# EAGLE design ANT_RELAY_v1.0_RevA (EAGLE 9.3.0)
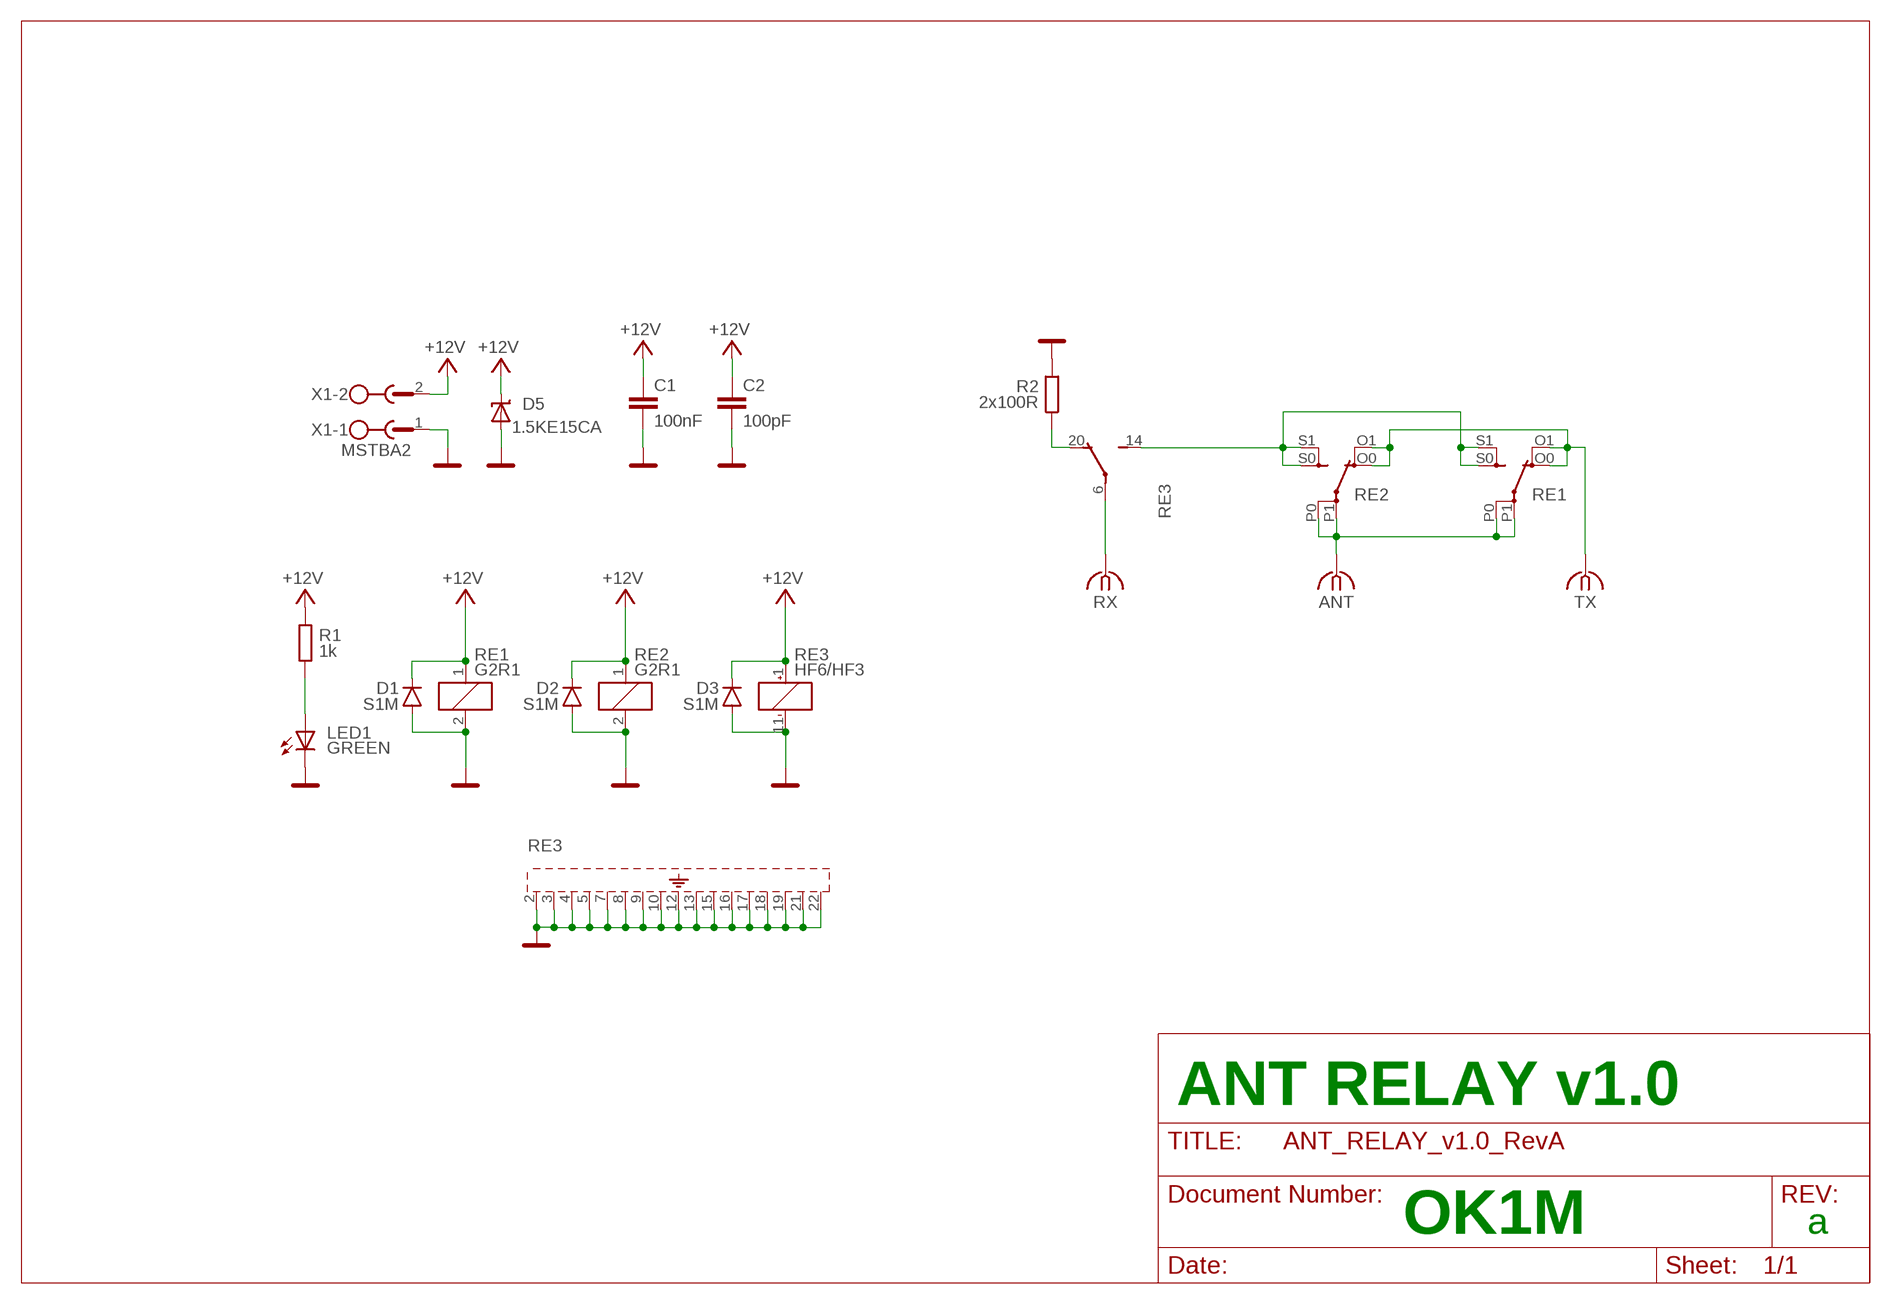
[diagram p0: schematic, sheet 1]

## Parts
ANT  N-180  [N-180]
C1  100nF  C-EUC0805  [C0805]
C2  100pF  C-EUC0805  [C0805]
D1  S1M  [SMA]
D2  S1M  [SMA]
D3  S1M  [SMA]
D5  1.5KE15CA  TRANSILDO201-15  [DO201-15]
LED1  GREEN  LED3MM  [LED3MM]
R1  1k  R-EU_M0805  [M0805]
R2  2x100R  R-EU_M1206  [M1206]
RE1  G2R1  G2RE  [G2RE]
RE2  G2R1  G2RE  [G2RE]
RE3  HF6/HF3  HF6-56+  [HF6-56]
RX  N-180  [N-180]
TX  N-180  [N-180]
X1  MSTBA2  [MSTBA2]

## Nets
+12V: C1.1 C2.1 D1.C D2.C D3.C D5.C R1.2 RE1.1 RE2.1 RE3.1 X1.2
ANT: ANT.1 RE1.P0(2:P) RE1.P1(2:P) RE2.P0(2:P) RE2.P1(2:P)
GND: C1.2 C2.2 D1.A D2.A D3.A D5.A LED1.K(C) R2.2 RE1.2 RE2.2 RE3.2 RE3.3 RE3.4 RE3.5 RE3.7 RE3.8 RE3.9 RE3.10 RE3.11 RE3.12 RE3.13 RE3.15 RE3.16 RE3.17 RE3.18 RE3.19 RE3.21 RE3.22 X1.1
N$2: RE3.6 RX.1
N$5: R2.1 RE3.20
N$20: LED1.A R1.1
N$30: RE1.S0(2:S) RE1.S1(2:S) RE2.S0(2:S) RE2.S1(2:S) RE3.14
TX: RE1.O0(2:O) RE1.O1(2:O) RE2.O0(2:O) RE2.O1(2:O) TX.1

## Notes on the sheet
- ANT RELAY v1.0
- OK1M | a

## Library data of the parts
ANT RX TX = #my:N-180
C1 C2 = rcl:C-EU: CAPACITOR, European symbol; SPICEPREFIX: C
D1-D3 = diode:S1M
D5 = #Marek:TRANSIL: TRANSIL
LED1 = led:LED: LED
R1 R2 = rcl:R-EU_: RESISTOR, European symbol
RE1 RE2 = relay:G2RE: RELAY 1 x switch, high current, Omron; OC_FARNELL: unknown; OC_NEWARK: unknown
RE3 = #hf6-56:HF6-56+
X1 = con-phoenix-508:MSTBA2: PHOENIX; MF: FARNELL; MPN: 1757242; OC_FARNELL: 3705171; OC_NEWARK: 71C4161

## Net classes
0 default: width 0.203 mm, drill 0.406 mm, clearance 0.203 mm

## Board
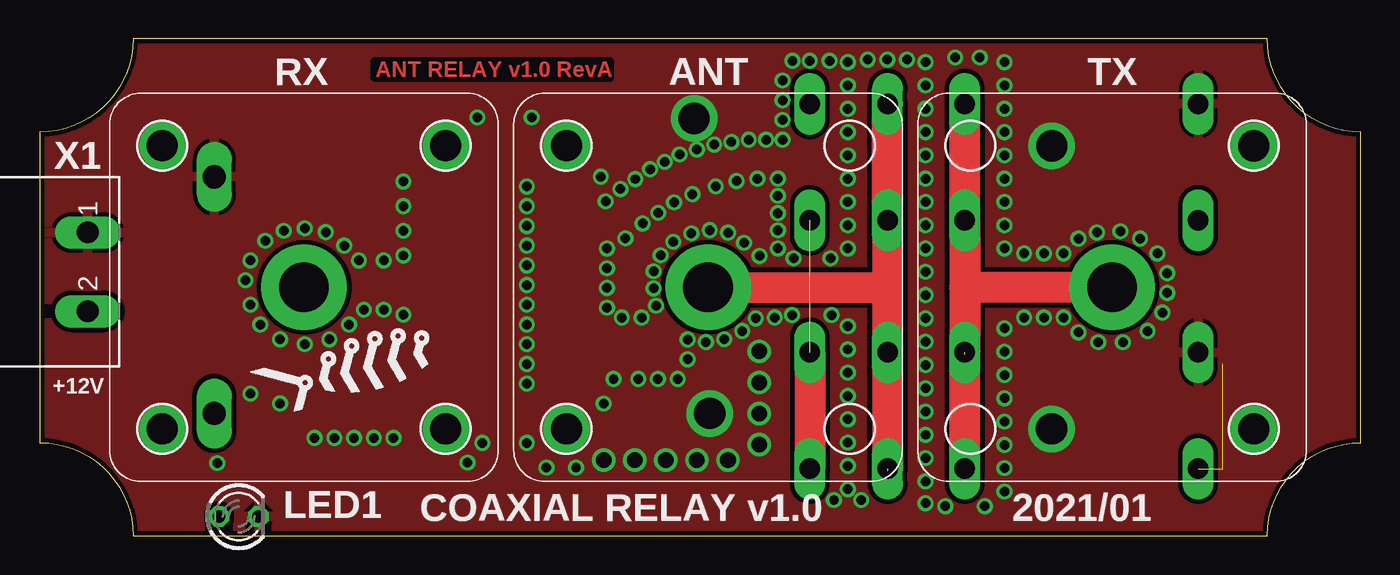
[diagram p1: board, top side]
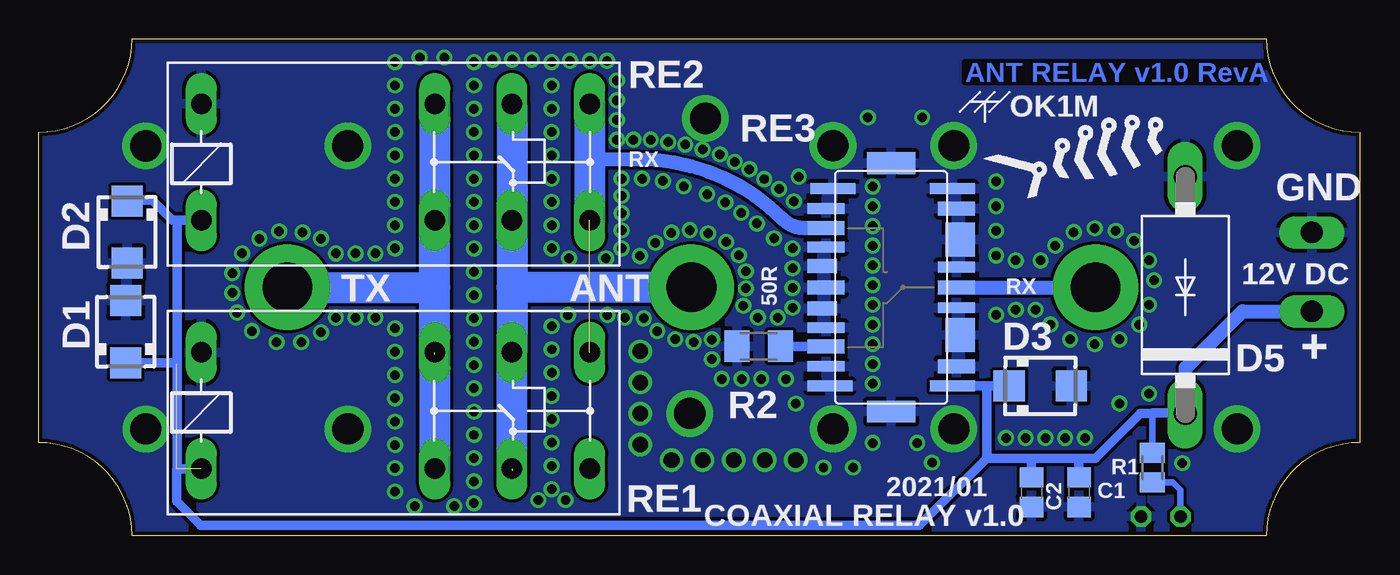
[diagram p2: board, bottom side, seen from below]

Size 85 x 32 mm. Coordinates in mm from the lower left corner, seen from the top.
Outline: 6,0 79,0 arc-90 85,6 85,26 arc-90 79,32 6,32 arc-90 0,26 0,6 arc-90 6,0
Copper layers (1*16): Top 0.035mm / dielectric 1.5mm / Bottom 0.035mm
Design rules "default *": minimum track width 10mil, minimum drill 24mil, track to track 8mil, track to pad 8mil, pad to pad 8mil, via to via 8mil, smd to smd 8mil, copper to edge 10mil, drill to drill 8mil, minimum pad ring 10mil, minimum via ring 8mil, stop-mask expansion 4mil, vias tented up to drill 0.7mm, thermal gap 10mil

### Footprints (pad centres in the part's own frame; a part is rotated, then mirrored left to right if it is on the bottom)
N-180 = drill 3.2 pad 5.5: 1 0,0
C0805 = smd 1.3 x 1.5: 1 -0.95,0; 2 0.95,0
SMA = smd 2 x 2: A 2,0; C -2,0
DO201-15 = drill 1.499 long: A 7.62,0; C -7.62,0
LED3MM = drill 0.813 octagon: A -1.27,0; K 1.27,0
M0805 = smd 1.3 x 1.6: 1 -0.95,0; 2 0.95,0
M1206 = smd 1.6 x 2: 1 -1.4,0; 2 1.4,0
G2RE = drill 1.321 long: 1 -2.54,-3.683; 2 -2.54,3.81; O0 12.471,-3.683; O1 12.471,3.81; P0 17.45,-3.683; P1 17.45,3.81; S0 22.454,-3.683; S1 22.454,3.81
HF6-56 = smd 0.7 x 2.9: 1 -6.35,-3.95; 11 6.35,-3.95; 12 6.35,3.75; 22 -6.35,3.95 | smd 0.9 x 2.4: 2 -5.08,-4.2; 6 0,-4.2; 10 5.08,-4.2; 14 3.81,4.2; 17 0,4.2; 20 -3.81,4.2 | smd 2.2 x 1.9: 3 -3.075,-4.45; 8 3.075,-4.45 | smd 1.4 x 3.1: 4 -8,0; 9 8,0 | smd 0.7 x 2.4: 5 -1.317,-4.2; 7 1.317,-4.2; 13 5.08,4.2; 15 2.6,4.2; 19 -2.6,4.2; 21 -5.08,4.2 | smd 0.9 x 1.9: 16 1.375,4.45; 18 -1.375,4.45
MSTBA2 = drill 1.397 long: 1 -2.54,5.08; 2 2.54,5.08

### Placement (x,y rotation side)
ANT  43,16 0 top
C1  18.06,2.81 270 bottom
C2  21.12,2.81 270 bottom
D1  79.41,13.14 90 bottom
D2  79.32,19.56 270 bottom
D3  20.56,9.65 0 bottom
D5  11.22,15.5 90 bottom
LED1  12.8,1.24 0 top
R1  13.34,4.39 90 bottom
R2  38.67,12.21 180 bottom
RE1  72,8 0 bottom
RE2  72,24 0 bottom
RE3  30.15,16 90 bottom
RX  17,16 0 top
TX  69,16 0 top
U$1  [RYBICKA_12MM]  20.95,10.79 0 top
U$2  [RYBICKA_12MM]  16.75,24.53 0 bottom
X1  -2,17 270 top

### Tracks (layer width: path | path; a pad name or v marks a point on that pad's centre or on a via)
+12V  (2 unrouted)
  Bottom 0.406: R1.2 13.34,7.87 13.34,7.88 | D5.C 11.25,7.91 13.3,7.91
  Bottom 0.61: RE3.1 24,9.65 | 24,9.65 D3.C | RE2.1 76.09,20.32 | 76.09,20.32 76.4,20.32 77.71,21.62 D2.C | RE1.1 76.09,4.32 76.09,20.32 | D1.C 76.2,11.14 76.12,11.06 | 24,9.65 24,5 | 18.1,5 17,5 14.12,7.88 13.34,7.88 13.3,7.91 11.19,7.91 | 18.1,5 21.27,5 | 21.27,5 24,5 | 24,5 28.32,0.68 74.57,0.68 76.12,2.23 76.12,4.32 | C1.1 18.06,4.96 18.1,5 | C2.1 21.12,4.84 21.27,5
  Bottom 0.9: 11.19,7.91 11.19,10.81 7.54,14.46 X1.2
ANT  (1 unrouted)
  Top 2: 54.55,16 RE2.P0 RE2.P1 | 54.55,16 RE1.P1 RE1.P0 | ANT.1 54.55,16
  Bottom 2: 54.55,16 54.55,20.19 RE2.P0 54.55,27.68 | 54.55,16 RE1.P1 | 54.55,16 ANT.1 54.55,16 | 54.55,4.19 54.55,11.68
GND  (via drill 0.61, 1, 2)
  other vias: 57,29 57,30.5 57,27.5 57,26 57,24.5 57,23 57,21.5 57,20 57,18.5 57,17 57,15.5 57,14 57,12.5 57,11 57,9.5 57,8 57,6.5 57,5 57,3.5 57,2.1 52,29 52,30.5 52,27.5 52,26 52,24.5 52,23 52,21.5 52,20 52,18.5 47.5,18.5 46.32,18.02 45.32,18.86 44.29,19.52 43.11,19.68 52,12 52,13.5 52,10.5 52,9 52,7.5 52,6 52,4.5 52,3 41.93,19.48 40.77,18.93 39.95,18.06 39.5,17.04 41.68,12.63 42.87,12.48 44.05,12.66 45.21,13.18 46.07,14 36.5,18.5 38.79,20.11 39.79,20.79 40.82,21.48 42,22 43.5,22.5 44.84,22.84 46.18,23 47.5,23 37.68,19.16 36.41,21.54 37.37,22.33 38.32,22.97 39.27,23.6 40.22,24.08 41.17,24.56 42.29,24.87 43.4,25.19 44.51,25.35 45.62,25.51 46.73,25.51 47.8,25.51 47.8,26.78 47.8,28.05 47.8,29.32 48.44,30.59 49.55,30.59 50.82,30.59 47.5,21.89 47.5,20.78 47.5,19.67 39.5,15.93 39.66,14.82 36.5,17.23 36.5,15.96 36.5,14.69 37.45,14.05 38.72,14.05 47.3,14.05 50.95,14.21 50.89,17.86 48.51,17.86 54.54,30.66 53.27,30.66 55.81,30.66 48.41,14.21 51.1,2.31 52.85,2.31 11.42,4.69 36.09,23.13 31.33,22.49 31.33,21.22 31.33,19.95 31.33,18.68 31.33,17.41 31.33,16.14 31.33,14.87 31.33,13.6 31.33,12.33 31.33,11.06 31.33,9.79 41.68,11.37 41.05,10.1 39.78,10.1 38.51,10.1 36.92,10.1 36.28,8.51 7.88,25.13 26.12,25.12 33.89,25.13 26.12,6.88 33.89,6.88 78.12,25.11 78.11,6.88 7.88,6.88 46.29,11.87 46.29,9.87 46.29,7.87 46.29,5.87 44.29,4.87 42.29,4.87 40.29,4.87 38.29,4.87 36.29,4.87 62.08,11.86 62.08,13.36 62.08,10.36 62.08,8.86 62.08,7.36 62.08,5.86 62.08,4.36 62.08,2.85 62.08,29 62.08,30.5 62.08,27.5 62.08,26 62.08,24.5 62.08,23 62.08,21.5 62.08,20 62.08,18.5 63.35,18.18 65.89,18.18 64.62,18.18 63.35,14.05 64.62,14.05 65.89,14.05 66.84,13.1 68.11,12.47 69.7,12.47 71.29,13.18 72.24,14.37 72.56,15.64 72.56,16.91 71.92,18.18 70.81,19.14 69.54,19.61 68.03,19.53 66.84,19.14 60.81,1.9 58.27,1.9 60.49,30.8 58.91,30.8 28.16,26.94 31.65,26.94 23.39,22.81 23.39,21.22 23.39,19.64 23.39,18.05 23.39,14.24 22.12,17.73 20.54,17.73 19.59,18.68 18.39,19.56 17.05,19.79 15.7,19.64 14.51,19 13.55,17.73 13.23,16.46 13.55,14.87 14.19,13.6 15.46,12.65 17.05,12.33 18.63,12.65 19.9,13.6 20.86,14.55 22.12,14.55 22.76,6.3 21.49,6.3 20.22,6.3 18.95,6.3 17.68,6.3 13.55,9.16 15.46,8.52 31.33,5.98 28.48,5.98 27.52,4.71 32.6,4.39 34.51,4.39 65.12,25.11 65.11,6.88 43.11,7.88 42.11,26.88
  pour Bottom: 0,0 85,0 85,32 0,32
  pour Top (isolate 0.3): 0,0 85,0 85,32 0,32
N$2
  Bottom 0.9: RE3.6 RX.1
N$5
  Bottom 0.61: RE3.20 37.25,12.19 R2.1
N$20
  Bottom 0.406: LED1.A 11.53,2.95 12.02,3.44 R1.1
N$30  (1 unrouted)
  Top 2: RE1.S1 RE1.S0
  Bottom 0.9: 49.55,24.27 49.31,24.23 46.4,24.23 arc45 37.14,20.4 arc-45 35.73,19.81 RE3.14
  Bottom 2: RE2.S1 49.55,24.27 RE2.S0
TX  (1 unrouted)
  Top 2: 59.53,16 RE2.O0 RE2.O1 | 59.53,16 RE1.O1 RE1.O0 | TX.1 59.53,16
  Bottom 2: RE1.O1 59.53,16 | 59.53,16 59.53,20.19 RE2.O0 59.53,27.68 | TX.1 59.53,16 | 59.53,11.68 59.53,4.19

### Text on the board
Top: ANT RELAY v1.0 RevA
Bottom: ANT RELAY v1.0 RevA
tPlace: +12V | COAXIAL RELAY v1.0 | 2021/01
bPlace: OK1M | RX | GND | 50R | 12V DC | RX | ANT | TX | + | 2021/01 | COAXIAL RELAY v1.0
